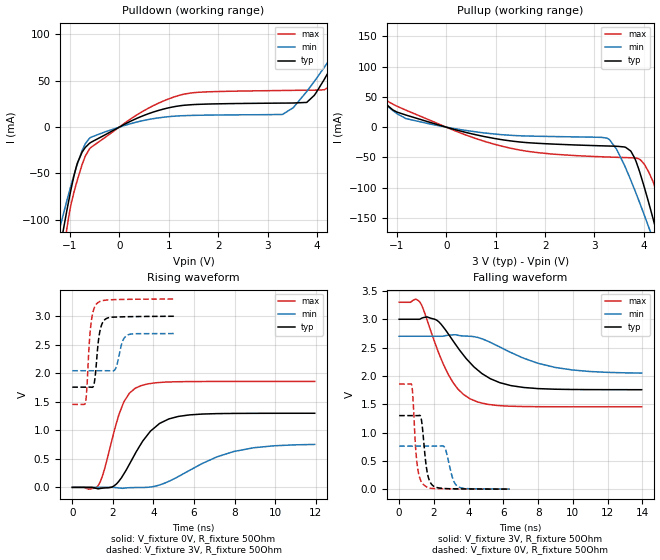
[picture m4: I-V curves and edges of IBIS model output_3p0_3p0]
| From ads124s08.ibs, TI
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|   output_3p0_3p0 Model
[Model]   output_3p0_3p0
Model_type   Output
Polarity   Non-Inverting
Vmeas = 1.5
Vref = 0
Cref = 2pF
Rref = 120
|   typ   min   max
|   (nom PVT)   (fast PVT)   (slow PVT)
C_comp   3.353e-12   3.122e-12   3.478e-12
| Where nom  PVT is Nominal Process, 3V, 27C
|   Fast PVT is Strong Process,  3.3V, -50C
|   Slow PVT is Weak Process,   2.7V, 125C
[Voltage Range]   3   2.7   3.3
|Junction Temperature
[Temperature Range]   27   125   -50
[Pullup Reference]   3   2.7   3.3
[Pulldown Reference]   0   0   0
[Power Clamp Reference]   3   2.7   3.3
[GND Clamp Reference]   0   0   0
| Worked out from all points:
|   slope of the pulldown table from 0 to 0.45 V, typ, clamps not added: 38.9 ohm
|   slope of the pullup table from 0 to 0.45 V, typ, clamps not added: 46.3 ohm
|   falling waveform, V_fixture 3V, R_fixture 50Ohm: 20-80 % time 2.15ns typ, 3.18ns min, 1.58ns max; typ from 3 V to 1.76 V
|   rising waveform, V_fixture 0V, R_fixture 50Ohm: 20-80 % time 1.45ns typ, 2.71ns min, 900ps max; typ from 0 V to 1.3 V
|   rising waveform, V_fixture 3V, R_fixture 50Ohm: 20-80 % time 225ps typ, 264ps min, 213ps max; typ from 1.76 V to 3 V
|   falling waveform, V_fixture 0V, R_fixture 50Ohm: 20-80 % time 284ps typ, 372ps min, 247ps max; typ from 1.3 V to 0.001 V
[Pulldown]
|   Voltage   I(typ)   I(min)   I(max)
-3V       -730.6mA   -547.9mA   -917.6mA
-1.205V   -131.2mA   -108.4mA   -163.2mA
-1.068V   -91.05mA   -80.12mA   -111mA
-848.1mV  -38.33mA   -39.27mA   -56.4mA
-609mV    -17.58mA   -12.18mA   -23.73mA
517.8mV   13.1mA     7.484mA    18.43mA
1.448V    24.19mA    12.63mA    36.89mA
3.303V    25.95mA    13.75mA    39.56mA
3.792V    26.69mA    38.39mA    39.86mA
4.283V    64.35mA    75.09mA    45.08mA
4.758V    111.4mA    112.5mA    100.9mA
6V        238.1mA    212.3mA    262.1mA
[Pullup]
|   Voltage   I(typ)   I(min)   I(max)
-3V       216.1mA    176.5mA    269mA
-1.73V    87.09mA    75.24mA    104.1mA
-1.272V   43.1mA     40.44mA    49.29mA
-815.7mV  19.97mA    14.07mA    28.02mA
1.171V    -21.32mA   -12.77mA   -32.42mA
3.237V    -31.12mA   -17.87mA   -49.32mA
3.445V    -31.6mA    -36.14mA   -49.9mA
3.735V    -39.57mA   -87.72mA   -50.62mA
4.095V    -124.1mA   -164.7mA   -73.79mA
4.24V     -168mA     -197.9mA   -104.3mA
4.392V    -215.7mA   -233.6mA   -158.8mA
6V        -757.1mA   -641.5mA   -830.3mA
[Ramp]
R_load = 50
|   typ   min   max
dV/dt_r   0.779437/1.45156e-09   0.456066/2.7537e-09   1.11395/9.00041e-10
dV/dt_f   0.746281/2.15027e-09   0.393815/3.23372e-09   1.10738/1.57573e-09
[Falling Waveform]
V_fixture = 3V
V_fixture_min = 2.7V
V_fixture_max = 3.3V
R_fixture = 50Ohm
|   Time   V(typ)   V(min)   V(max)
0s        3V         2.7V       3.3V
1.204ns   3.003V     2.7V       3.298V
2.18ns    2.98V      2.7V       2.484V
2.823ns   2.744V     2.718V     2.028V
3.369ns   2.503V     2.718V     1.772V
4.074ns   2.235V     2.7V       1.596V
5.24ns    1.952V     2.593V     1.493V
6.431ns   1.829V     2.413V     1.465V
8.955ns   1.765V     2.151V     1.455V
13.96ns   1.756V     2.05V      1.454V
[Rising Waveform]
V_fixture = 0V
V_fixture_min = 0V
V_fixture_max = 0V
R_fixture = 50Ohm
|   Time   V(typ)   V(min)   V(max)
0s        1.561nV    2.225nV    1.411nV
1.268ns   -24.4mV    -2.675uV   27.13mV
1.59ns    -10.09mV   13.78uV    320.6mV
2.061ns   26.4mV     -1.133mV   978.1mV
2.542ns   236mV      -14.1mV    1.499V
3.369ns   750.2mV    -2.745mV   1.78V
4.304ns   1.12V      41.91mV    1.838V
5.24ns    1.244V     191.9mV    1.851V
7.955ns   1.296V     627.9mV    1.856V
11.96ns   1.299V     752.6mV    1.857V
[Rising Waveform]
V_fixture = 3V
V_fixture_min = 2.7V
V_fixture_max = 3.3V
R_fixture = 50Ohm
|   Time   V(typ)   V(min)   V(max)
0s        1.756V     2.044V     1.454V
633.6ps   1.756V     2.044V     1.465V
913.7ps   1.756V     2.044V     2.839V
1.086ns   1.832V     2.044V     3.146V
1.204ns   2.242V     2.044V     3.218V
1.39ns    2.78V      2.044V     3.26V
1.669ns   2.956V     2.044V     3.281V
2.129ns   2.984V     2.076V     3.29V
2.752ns   2.99V      2.673V     3.295V
5.064ns   2.998V     2.695V     3.299V
[Falling Waveform]
V_fixture = 0V
V_fixture_min = 0V
V_fixture_max = 0V
R_fixture = 50Ohm
|   Time   V(typ)   V(min)   V(max)
0s        1.299V     760.1mV    1.857V
716.8ps   1.299V     760.1mV    1.844V
1.028ns   1.299V     760.1mV    457mV
1.258ns   1.264V     760.1mV    142.1mV
1.413ns   845.9mV    760.1mV    77.11mV
1.625ns   277.9mV    760.1mV    34.82mV
1.972ns   55.64mV    760mV      12.39mV
2.6ns     13.09mV    746.8mV    6.759mV
3.4ns     5.883mV    44.18mV    3.852mV
6.356ns   1.251mV    2.872mV    588.4uV
